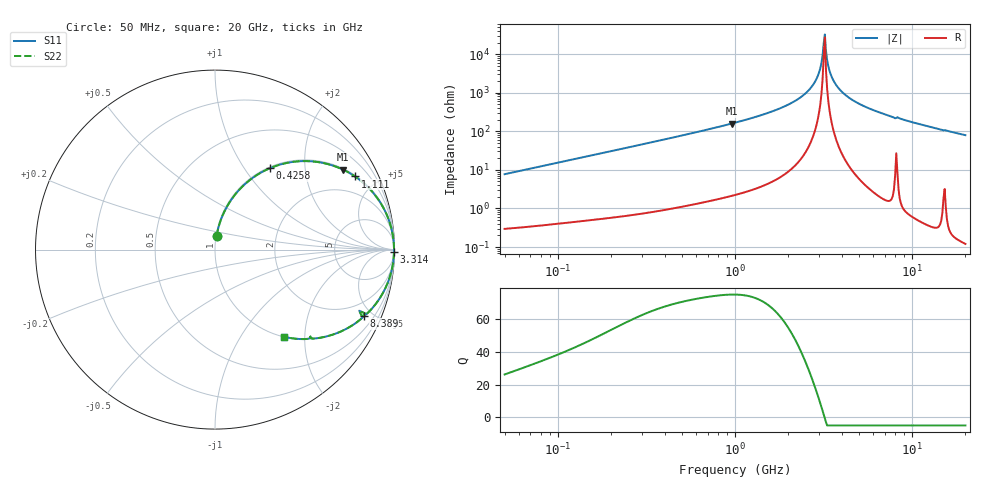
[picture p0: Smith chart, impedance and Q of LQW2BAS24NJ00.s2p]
!Murata Part Number: LQW2BAS24NJ00
!These Parameters are Measured in Series Mode Connection
!  o--[Z]--o
!Port1  Port2
!  o-------o
!Freq. Start=50[MHz] Stop=20[GHz], 401[Steps]
# Hz S RI R 50
!Freq.(Hz) S11(Real) S11(Imag) S21(Real) S21(Imag) S12(Real) S12(Imag) S22(Real) S22(Imag)
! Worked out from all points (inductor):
!   401 points, 50 MHz to 20 GHz, reference 50 ohm
!   read as one part in series: L = 24.5 nH near 51.52 MHz
!   highest Q = 74.9 at 956.1 MHz (marker M1), where L = 26.3 nH
!   self-resonance near 3.169 GHz
!   S11 on the Smith chart (normalised r, x): 50 MHz: 1.01, +0.15; 425.8 MHz: 1.02, +1.31; 1.111 GHz: 1.05, +3.80; 3.314 GHz: open; 8.389 GHz: 1.06, -4.45; 20 GHz: 1.00, -1.59
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5e7  0.00882 0.0763  0.9912 -0.0763  0.9912 -0.0763  0.00882 0.0763
1.364002e8  0.0459 0.1983  0.9541 -0.1983  0.9541 -0.1983  0.0459 0.1983
3.721004e8  0.25 0.4255  0.75 -0.4255  0.75 -0.4255  0.25 0.4255
4.258008e8  0.3042 0.4528  0.6958 -0.4528  0.6958 -0.4528  0.3042 0.4528
9.560587e8  0.7121 0.4462  0.2879 -0.4462  0.2879 -0.4462  0.7121 0.4462
1e9  0.7334 0.4356  0.2666 -0.4356  0.2666 -0.4356  0.7334 0.4356
1.110545e9  0.7803 0.4074  0.2197 -0.4074  0.2197 -0.4074  0.7803 0.4074
1.99176e9  0.9564 0.1953  0.0436 -0.1953  0.0436 -0.1953  0.9564 0.1953
2.383959e9  0.9817 0.1219  0.0183 -0.1219  0.0183 -0.1219  0.9817 0.1219
2.728004e9  0.9927 0.0664  0.00733 -0.0664  0.00733 -0.0664  0.9927 0.0664
2.98453e9  0.9964 0.0293  0.00358 -0.0293  0.00358 -0.0293  0.9964 0.0293
3.168813e9  0.9974 0.00455  0.00264 -0.00455  0.00264 -0.00455  0.9974 0.00455
3.265178e9  0.9974 -0.00785  0.00264 0.00785  0.00264 0.00785  0.9974 -0.00785
3.314454e9  0.9972 -0.014  0.00275 0.014  0.00275 0.014  0.9972 -0.014
3.415248e9  0.9968 -0.0264  0.00322 0.0264  0.00322 0.0264  0.9968 -0.0264
3.519108e9  0.996 -0.0388  0.00399 0.0388  0.00399 0.0388  0.996 -0.0388
4.087748e9  0.9874 -0.1008  0.0126 0.1008  0.0126 0.1008  0.9874 -0.1008
5.194772e9  0.9562 -0.1996  0.0438 0.1996  0.0438 0.1996  0.9562 -0.1996
7.442007e9  0.862 -0.3418  0.138 0.3418  0.138 0.3418  0.862 -0.3418
8.389408e9  0.8284 -0.3702  0.1716 0.3702  0.1716 0.3702  0.8284 -0.3702
1.276073e10  0.6248 -0.4829  0.3752 0.4829  0.3752 0.4829  0.6248 -0.4829
2e10  0.3869 -0.4863  0.6131 0.4863  0.6131 0.4863  0.3869 -0.4863
